|   stm32f0_440_lqfp64 IBIS Model
[IBIS ver]   4.2
[File name]  stm32f0_440_lqfp64.ibs
[File Rev]   1.0
[Date]   15-5-2013
[Source] Data Created at STMicroelectronics
[Notes]   File originated from ELDO simulations.
[Disclaimer]  This information is for modeling purpose only and is
   not guaranted. The information is subject to change without
   notice.
[Copyright] Copyright 2015 STMicroelectronics Inc.
[Component] stm32f0_440_lqfp64
[Manufacturer] STMicroelectronics
[Package]
| variable   typ   min   max
R_pkg   0.0   NA   NA
L_pkg   0.0H   NA   NA
C_pkg   0.0F   NA   NA
[Pin] signal_name  model_name   R_pin   L_pin   C_pin
1   VBAT  POWER   69.0E-3   4.2E-9   120.0E-15
2   PC13  io8p_sudq_tc   63.8E-3   3.7E-9   93.5E-15
3   PC14  io8p_sudq_tc   59.3E-3   3.2E-9   71.0E-15
4   PC15  io8p_sudq_tc   55.7E-3   2.8E-9   52.7E-15
5   PF0   io8p_sudq_ft   52.9E-3   2.6E-9   38.4E-15
6   PF1   io8p_sudq_ft   50.9E-3   2.3E-9   28.2E-15
7   NRST  ioreset_tc_v33   49.7E-3   2.2E-9   22.0E-15
8   PC0   io8p_sudq_ft   49.3E-3   2.2E-9   20.0E-15
9   PC1   io8p_sudq_ft   49.3E-3   2.2E-9   20.0E-15
10   PC2   io8p_sudq_ft   49.7E-3   2.2E-9   22.0E-15
11   PC3   io8p_sudq_ft   50.9E-3   2.3E-9   28.2E-15
12   VSSA  GND   52.9E-3   2.6E-9   38.4E-15
13   VDDA  POWER   55.7E-3   2.8E-9   52.7E-15
14   PA0   io8p_sudq_ft   59.3E-3   3.2E-9   71.0E-15
15   PA1   io8p_sudq_ft   63.8E-3   3.7E-9   93.5E-15
16   PA2   io8p_sudq_ft   69.0E-3   4.2E-9   120.0E-15
17   PA3   io8p_sudq_ft   69.0E-3   4.2E-9   120.0E-15
18   PF4   io8p_sudq_ft   63.8E-3   3.7E-9   93.5E-15
19   PF5   io8p_sudq_ft   59.3E-3   3.2E-9   71.0E-15
20   PA4   io8p_sudq_ft   55.7E-3   2.8E-9   52.7E-15
21   PA5   io8p_sudq_ft   52.9E-3   2.6E-9   38.4E-15
22   PA6   io8p_sudq_ft   50.9E-3   2.3E-9   28.2E-15
23   PA7   io8p_sudq_ft   49.7E-3   2.2E-9   22.0E-15
24   PC4   io8p_sudq_ft   49.3E-3   2.2E-9   20.0E-15
25   PC5   io8p_sudq_ft   49.3E-3   2.2E-9   20.0E-15
26   PB0   io8p_sudq_ft   49.7E-3   2.2E-9   22.0E-15
27   PB1   io8p_sudq_ft   50.9E-3   2.3E-9   28.2E-15
28   PB2   io8p_sudq_ft   52.9E-3   2.6E-9   38.4E-15
29   PB10  io8p_sudq_i2cin_lv_ft   55.7E-3   2.8E-9   52.7E-15
30   PB11  io8p_sudq_i2cin_lv_ft   59.3E-3   3.2E-9   71.0E-15
31   VSS   GND   63.8E-3   3.7E-9   93.5E-15
32   VDD   POWER   69.0E-3   4.2E-9   120.0E-15
33   PB12  io8p_sudq_ft   69.0E-3   4.2E-9   120.0E-15
34   PB13  io8p_sudq_ft   63.8E-3   3.7E-9   93.5E-15
35   PB14  io8p_sudq_ft   59.3E-3   3.2E-9   71.0E-15
36   PB15  io8p_sudq_ft   55.7E-3   2.8E-9   52.7E-15
37   PC6   io8p_sudq_ft   52.9E-3   2.6E-9   38.4E-15
38   PC7   io8p_sudq_ft   50.9E-3   2.3E-9   28.2E-15
39   PC8   io8p_sudq_ft   49.7E-3   2.2E-9   22.0E-15
40   PC9   io8p_sudq_ft   49.3E-3   2.2E-9   20.0E-15
41   PA8   io8p_sudq_ft   49.3E-3   2.2E-9   20.0E-15
42   PA9   io8p_sudq_ft   49.7E-3   2.2E-9   22.0E-15
43   PA10  io8p_sudq_ft   50.9E-3   2.3E-9   28.2E-15
44   PA11  io8p_sudq_ft   52.9E-3   2.6E-9   38.4E-15
45   PA12  io8p_sudq_ft   55.7E-3   2.8E-9   52.7E-15
46   PA13  io8p_sudq_ft   59.3E-3   3.2E-9   71.0E-15
47   PF6   io8p_sudq_i2cin_lv_ft   63.8E-3   3.7E-9   93.5E-15
48   PF7   io8p_sudq_i2cin_lv_ft   69.0E-3   4.2E-9   120.0E-15
49   PA14  io8p_sudq_ft   69.0E-3   4.2E-9   120.0E-15
50   PA15  io8p_sudq_ft   63.8E-3   3.7E-9   93.5E-15
51   PC10  io8p_sudq_ft   59.3E-3   3.2E-9   71.0E-15
52   PC11  io8p_sudq_ft   55.7E-3   2.8E-9   52.7E-15
53   PC12  io8p_sudq_ft   52.9E-3   2.6E-9   38.4E-15
54   PD2   io8p_sudq_ft   50.9E-3   2.3E-9   28.2E-15
55   PB3   io8p_sudq_ft   49.7E-3   2.2E-9   22.0E-15
56   PB4   io8p_sudq_ft   49.3E-3   2.2E-9   20.0E-15
57   PB5   io8p_sudq_ft   49.3E-3   2.2E-9   20.0E-15
58   PB6   io8p_sudq_i2cin_lv_ft   49.7E-3   2.2E-9   22.0E-15
59   PB7   io8p_sudq_i2cin_lv_ft   50.9E-3   2.3E-9   28.2E-15
60   BOOT0 vpp_test_hv   52.9E-3   2.6E-9   38.4E-15
61   PB8   io8p_sudq_i2cin_lv_ft   55.7E-3   2.8E-9   52.7E-15
62   PB9   io8p_sudq_i2cin_lv_ft   59.3E-3   3.2E-9   71.0E-15
63   VSS   GND   63.8E-3   3.7E-9   93.5E-15
64   VDD   POWER   69.0E-3   4.2E-9   120.0E-15
[Model Selector] io8p_sudq_ft
io8p01_sudq_ft_pd_lv  "SPEED01 2P0V, PD=40kOhm"
io8p01_sudq_ft_pu_lv  "SPEED01 2P0V, PU=40kOhm"
io8p01_sudq_ft_lv  "SPEED01 2P0V"
io8p10_sudq_ft_pd_lv  "SPEED10 2P0V, PD=40kOhm"
io8p10_sudq_ft_pu_lv  "SPEED10 2P0V, PU=40kOhm"
io8p10_sudq_ft_lv  "SPEED10 2P0V"
io8p11_sudq_ft_pd_lv  "SPEED11 2P0V, PD=40kOhm"
io8p11_sudq_ft_pu_lv  "SPEED11 2P0V, PU=40kOhm"
io8p11_sudq_ft_lv  "SPEED11 2P0V"
io8p01_sudq_ft_pd  "SPEED01, PD=40kOhm"
io8p01_sudq_ft_pu  "SPEED01, PU=40kOhm"
io8p01_sudq_ft  "SPEED01"
io8p10_sudq_ft_pd  "SPEED10, PD=40kOhm"
io8p10_sudq_ft_pu  "SPEED10, PU=40kOhm"
io8p10_sudq_ft  "SPEED10"
io8p11_sudq_ft_pd  "SPEED11, PD=40kOhm"
io8p11_sudq_ft_pu  "SPEED11, PU=40kOhm"
io8p11_sudq_ft  "SPEED11"
[Model Selector] io8p_sudq_i2cin_lv_ft
io8p01_sudq_i2cin_lv_ft_pd_lv  "SPEED01 2P0V, PD=40kOhm"
io8p01_sudq_i2cin_lv_ft_pu_lv  "SPEED01 2P0V, PU=40kOhm"
io8p01_sudq_i2cin_lv_ft_lv  "SPEED01 2P0V"
io8p10_sudq_i2cin_lv_ft_pd_lv  "SPEED10 2P0V, PD=40kOhm"
io8p10_sudq_i2cin_lv_ft_pu_lv  "SPEED10 2P0V, PU=40kOhm"
io8p10_sudq_i2cin_lv_ft_lv  "SPEED10 2P0V"
io8p11_sudq_i2cin_lv_ft_pd_lv  "SPEED11 2P0V, PD=40kOhm"
io8p11_sudq_i2cin_lv_ft_pu_lv  "SPEED11 2P0V, PU=40kOhm"
io8p11_sudq_i2cin_lv_ft_lv  "SPEED11 2P0V"
io8p01_sudq_i2cin_lv_ft_pd  "SPEED01, PD=40kOhm"
io8p01_sudq_i2cin_lv_ft_pu  "SPEED01, PU=40kOhm"
io8p01_sudq_i2cin_lv_ft  "SPEED01"
io8p10_sudq_i2cin_lv_ft_pd  "SPEED10, PD=40kOhm"
io8p10_sudq_i2cin_lv_ft_pu  "SPEED10, PU=40kOhm"
io8p10_sudq_i2cin_lv_ft  "SPEED10"
io8p11_sudq_i2cin_lv_ft_pd  "SPEED11, PD=40kOhm"
io8p11_sudq_i2cin_lv_ft_pu  "SPEED11, PU=40kOhm"
io8p11_sudq_i2cin_lv_ft  "SPEED11"
[Model Selector] io8p_sudq_tc
io8p01_sudq_tc_pd_lv  "SPEED01 2P0V, PD=40kOhm"
io8p01_sudq_tc_pu_lv  "SPEED01 2P0V, PU=40kOhm"
io8p01_sudq_tc_lv  "SPEED01 2P0V"
io8p10_sudq_tc_pd_lv  "SPEED10 2P0V, PD=40kOhm"
io8p10_sudq_tc_pu_lv  "SPEED10 2P0V, PU=40kOhm"
io8p10_sudq_tc_lv  "SPEED10 2P0V"
io8p11_sudq_tc_pd_lv  "SPEED11 2P0V, PD=40kOhm"
io8p11_sudq_tc_pu_lv  "SPEED11 2P0V, PU=40kOhm"
io8p11_sudq_tc_lv  "SPEED11 2P0V"
io8p01_sudq_tc_pd  "SPEED01, PD=40kOhm"
io8p01_sudq_tc_pu  "SPEED01, PU=40kOhm"
io8p01_sudq_tc  "SPEED01"
io8p10_sudq_tc_pd  "SPEED10, PD=40kOhm"
io8p10_sudq_tc_pu  "SPEED10, PU=40kOhm"
io8p10_sudq_tc  "SPEED10"
io8p11_sudq_tc_pd  "SPEED11, PD=40kOhm"
io8p11_sudq_tc_pu  "SPEED11, PU=40kOhm"
io8p11_sudq_tc  "SPEED11"
[Model Selector] ioreset_tc_v33
ioreset_tc_v33_pu_lv  "IORESET 2V + PU=40kOhm"
ioreset_tc_v33_nopu_lv  "IORESET 2V"
ioreset_tc_v33_pu  "IORESET + PU=40kOhm"
ioreset_tc_v33_nopu  "IORESET"
[Model Selector] vpp_test_hv
vpp_test_hv_3p3  "Input Buffer"
vpp_test_hv_2p4  "Input Buffer 2P0V"
| Models and submodels in the file (60): io8p01_sudq_ft_pd_lv (I/O), io8p01_sudq_ft_pu_lv (I/O), io8p01_sudq_ft_lv (I/O), io8p10_sudq_ft_pd_lv (I/O), io8p10_sudq_ft_pu_lv (I/O), io8p10_sudq_ft_lv (I/O), io8p11_sudq_ft_pd_lv (I/O), io8p11_sudq_ft_pu_lv (I/O), io8p11_sudq_ft_lv (I/O), io8p01_sudq_ft_pd (I/O), io8p01_sudq_ft_pu (I/O), io8p01_sudq_ft (I/O), io8p10_sudq_ft_pd (I/O), io8p10_sudq_ft_pu (I/O), io8p10_sudq_ft (I/O), io8p11_sudq_ft_pd (I/O), io8p11_sudq_ft_pu (I/O), io8p11_sudq_ft (I/O), io8p01_sudq_i2cin_lv_ft_pd_lv (I/O), io8p01_sudq_i2cin_lv_ft_pu_lv (I/O), io8p01_sudq_i2cin_lv_ft_lv (I/O), io8p10_sudq_i2cin_lv_ft_pd_lv (I/O), io8p10_sudq_i2cin_lv_ft_pu_lv (I/O), io8p10_sudq_i2cin_lv_ft_lv (I/O), io8p11_sudq_i2cin_lv_ft_pd_lv (I/O), io8p11_sudq_i2cin_lv_ft_pu_lv (I/O), io8p11_sudq_i2cin_lv_ft_lv (I/O), io8p01_sudq_i2cin_lv_ft_pd (I/O), io8p01_sudq_i2cin_lv_ft_pu (I/O), io8p01_sudq_i2cin_lv_ft (I/O), io8p10_sudq_i2cin_lv_ft_pd (I/O), io8p10_sudq_i2cin_lv_ft_pu (I/O), io8p10_sudq_i2cin_lv_ft (I/O), io8p11_sudq_i2cin_lv_ft_pd (I/O), io8p11_sudq_i2cin_lv_ft_pu (I/O), io8p11_sudq_i2cin_lv_ft (I/O), io8p01_sudq_tc_pd_lv (I/O), io8p01_sudq_tc_pu_lv (I/O), io8p01_sudq_tc_lv (I/O), io8p10_sudq_tc_pd_lv (I/O), io8p10_sudq_tc_pu_lv (I/O), io8p10_sudq_tc_lv (I/O), io8p11_sudq_tc_pd_lv (I/O), io8p11_sudq_tc_pu_lv (I/O), io8p11_sudq_tc_lv (I/O), io8p01_sudq_tc_pd (I/O), io8p01_sudq_tc_pu (I/O), io8p01_sudq_tc (I/O), io8p10_sudq_tc_pd (I/O), io8p10_sudq_tc_pu (I/O), io8p10_sudq_tc (I/O), io8p11_sudq_tc_pd (I/O), io8p11_sudq_tc_pu (I/O), io8p11_sudq_tc (I/O), ioreset_tc_v33_pu_lv (I/O_open_drain), ioreset_tc_v33_nopu_lv (I/O_open_drain), ioreset_tc_v33_pu (I/O_open_drain), ioreset_tc_v33_nopu (I/O_open_drain), vpp_test_hv_2p4 (Input), vpp_test_hv_3p3 (Input)
